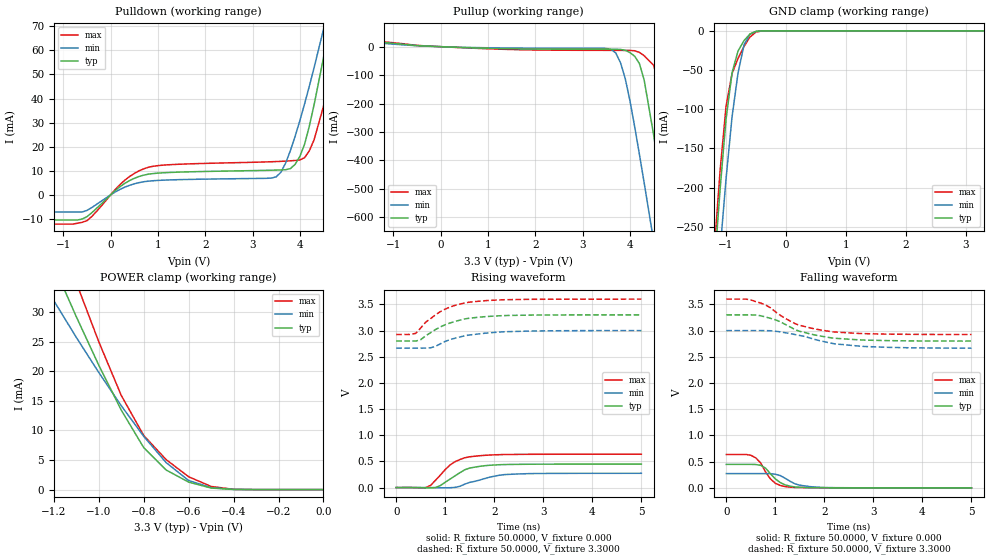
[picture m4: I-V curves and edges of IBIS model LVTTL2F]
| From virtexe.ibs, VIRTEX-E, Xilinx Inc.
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|   Model LVTTL2F
[Model]   LVTTL2F
Model_type   I/O
Polarity   Non-Inverting
Enable   Active-Low
Vinl =   0.800V
Vinh =   2.000V
Vmeas =   1.4000V
Cref =  35.0000pF
Rref =   1.0000M
Vref =  0.000V
C_comp   5.0000pF   4.0000pF   6.0000pF
[Temperature Range]   25.0000   100.0000   0.000
[Voltage Range]   3.3000V   3.0000V   3.6000V
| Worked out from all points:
|   slope of the pulldown table from 0 to 0.495 V, typ, clamps not added: 72.6 ohm
|   slope of the pullup table from 0 to 0.495 V, typ, clamps not added: 152 ohm
|   GND clamp passes 1 mA (typ) near -0.51 V on its own axis
|   POWER clamp passes 1 mA (typ) near -0.57 V on its own axis
|   rising waveform, R_fixture 50.0000, V_fixture 0.000: 20-80 % time 474ps typ, 633ps min, 448ps max; typ from 0 V to 0.448 V
|   rising waveform, R_fixture 50.0000, V_fixture 3.3000: 20-80 % time 705ps typ, 783ps min, 640ps max; typ from 2.8 V to 3.3 V
|   falling waveform, R_fixture 50.0000, V_fixture 0.000: 20-80 % time 309ps typ, 354ps min, 286ps max; typ from 0.448 V to 0 V
|   falling waveform, R_fixture 50.0000, V_fixture 3.3000: 20-80 % time 876ps typ, 1.04ns min, 829ps max; typ from 3.3 V to 2.8 V
[Pulldown]
| voltage   I(typ)   I(min)   I(max)
-3.3V     -10.44mA   -7.098mA   -12.15mA
-700mV    -10.44mA   -7.098mA   -11.78mA
300mV     4.77mA     3.204mA    6.092mA
800mV     8.599mA    5.7mA      11.47mA
3.5V      10.29mA    7.484mA    13.84mA
3.7V      10.45mA    13.24mA    14.02mA
4V        15.95mA    30.8mA     14.5mA
4.2V      28.48mA    45.11mA    18.27mA
4.5V      56.99mA    68.77mA    36.77mA
4.7V      78.21mA    85.56mA    59.04mA
4.9V      100.4mA    103mA      84.05mA
6.6V      305.2mA    264.8mA    320.6mA
[Pullup]
| voltage   I(typ)   I(min)   I(max)
-3.3V     57.9mA     57mA       55.1mA
-500mV    3.885mA    3.024mA    4.653mA
3.6V      -9.158mA   -9.435mA   -13.01mA
3.7V      -9.22mA    -22.12mA   -13.04mA
3.9V      -12.77mA   -112.2mA   -13.12mA
4.2V      -59.66mA   -379.1mA   -20.13mA
4.3V      -117.2mA   -478.9mA   -31.66mA
4.5V      -309.9mA   -683.4mA   -65.4mA
4.7V      -530mA     -891.4mA   -185.2mA
4.9V      -757.3mA   -1.101A    -399.7mA
5.1V      -988.1mA   -1.313A    -630.8mA
6.6V      -2.753A    -2.919A    -2.443A
[GND_clamp]
| voltage   I(typ)   I(min)   I(max)
-3.3V     -2.749A    -2.594A    -2.804A
-1.2V     -306mA     -377.1mA   -282.7mA
-1.1V     -202.5mA   -280mA     -178.8mA
-1V       -112.5mA   -188.5mA   -95.98mA
-900mV    -53.5mA    -109.7mA   -54.53mA
-800mV    -25.67mA   -53.59mA   -35.13mA
-700mV    -12.44mA   -17.88mA   -19.82mA
-600mV    -3.982mA   -4.202mA   -7.865mA
-500mV    -601.5uA   -800.3uA   -1.508mA
-400mV    -51.05uA   -119.3uA   -124.3uA
3.3V      18.74nA    3.634uA    18.92nA
[POWER_clamp]
| voltage   I(typ)   I(min)   I(max)
-3.3V     237mA      175.9mA    284.4mA
-1.3V     46.69mA    38.29mA    56.33mA
-1.2V     37.79mA    31.9mA     45.45mA
-1.1V     29.2mA     25.71mA    34.95mA
-1V       21.01mA    19.78mA    24.97mA
-900mV    13.43mA    14.17mA    15.91mA
-800mV    7.091mA    8.993mA    9.139mA
-700mV    3.305mA    4.554mA    5.052mA
-600mV    1.265mA    1.529mA    2.172mA
-500mV    263.8uA    333.6uA    531.5uA
-400mV    22.63uA    44.12uA    49.77uA
0V        18.8nA     38.36nA    22.53nA
[Ramp]
| variable   typ   min   max
dV/dt_r   0.2686/0.4938n   0.1635/0.6138n   0.3821/0.4399n
dV/dt_f   0.3000/0.8729n   0.2010/1.0262n   0.4050/0.8198n
R_load = 50.0000
[Rising Waveform]
R_fixture = 50.0000
V_fixture = 0.000
| time   V(typ)   V(min)   V(max)
0s        4.622uV    5uV        4.595uV
600ps     -5.447mV   17.29uV    -2.556mV
700ps     -5.85mV    -503.8uV   40.9mV
800ps     -785.5uV   -2.113mV   137.4mV
1.1ns     162.9mV    -3.09mV    431.9mV
1.3ns     284.3mV    24.05mV    535.7mV
1.5ns     373.1mV    98.9mV     587.9mV
2ns       430.9mV    217.2mV    624.7mV
2.3ns     441mV      252mV      631.9mV
5ns       447.7mV    272.5mV    636.8mV
[Rising Waveform]
R_fixture = 50.0000
V_fixture = 3.3000
V_fixture_min = 3.0000
V_fixture_max = 3.6000
| time   V(typ)   V(min)   V(max)
0s        2.799V     2.664V     2.925V
400ps     2.799V     2.664V     2.947V
500ps     2.826V     2.664V     3.05V
600ps     2.899V     2.665V     3.159V
700ps     2.958V     2.67V      3.226V
900ps     3.07V      2.746V     3.361V
1.2ns     3.175V     2.854V     3.481V
1.5ns     3.237V     2.916V     3.543V
2.6ns     3.292V     2.987V     3.595V
5ns       3.3V       2.999V     3.6V
[Falling Waveform]
R_fixture = 50.0000
V_fixture = 0.000
| time   V(typ)   V(min)   V(max)
0s        447.8mV    272.6mV    636.8mV
400ps     447.8mV    272.6mV    637.2mV
600ps     445.4mV    272.6mV    572.2mV
700ps     429.5mV    272.7mV    476.4mV
800ps     376.8mV    272.7mV    302mV
900ps     268.5mV    270.7mV    170.5mV
1.2ns     56.78mV    182.8mV    24.31mV
1.5ns     10.45mV    50.78mV    5.413mV
1.9ns     2.943mV    10.97mV    1.792mV
5ns       62.97uV    110.5uV    45.59uV
[Falling Waveform]
R_fixture = 50.0000
V_fixture = 3.3000
V_fixture_min = 3.0000
V_fixture_max = 3.6000
| time   V(typ)   V(min)   V(max)
0s        3.3V       3V         3.6V
500ps     3.3V       3V         3.585V
800ps     3.259V     2.999V     3.488V
1ns       3.206V     2.988V     3.36V
1.2ns     3.119V     2.959V     3.233V
1.4ns     3.02V      2.924V     3.133V
1.7ns     2.938V     2.86V      3.054V
2.1ns     2.867V     2.767V     2.986V
2.8ns     2.819V     2.697V     2.942V
5ns       2.8V       2.665V     2.925V
